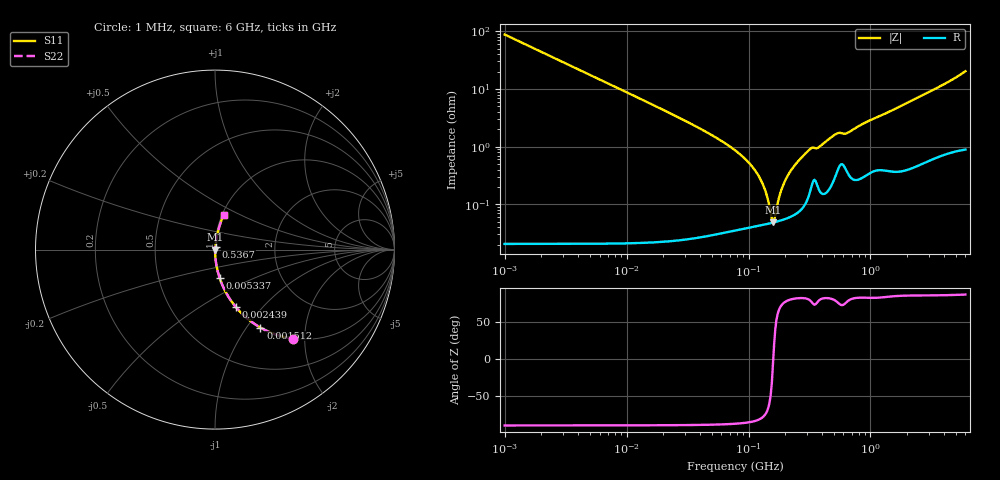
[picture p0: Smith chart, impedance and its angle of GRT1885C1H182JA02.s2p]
!Murata Part Number: GRT1885C1H182JA02
!These Parameters are Measured in Series Mode Connection
!Data Generated on Jun 19, 2026
!  o--ll--o
!Port1  Port2
!  o------o
!Operation Temp=25[degC], DC Bias Voltage=0[V]
!Freq. Start=1000[kHz] Stop=6[GHz] 401[Steps]
# Hz S RI R 50
!Freq.(Hz) S11(Real) S11(Imag) S21(Real) S21(Imag) S12(Real) S12(Imag) S22(Real) S22(Imag)
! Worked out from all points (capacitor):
!   401 points, 1 MHz to 6 GHz, reference 50 ohm
!   read as one part in series: C = 1.81 nF near 1.044 MHz
!   lowest |Z| = 48.4 mohm at 158.8 MHz (marker M1)
!   series resonance near 159.6 MHz, so ESL is about 550 pH
!   S11 on the Smith chart (normalised r, x): 1 MHz: 1.00, -1.76; 1.512 MHz: 1.00, -1.16; 2.439 MHz: 1.00, -0.72; 5.337 MHz: 1.00, -0.33; 536.7 MHz: 1.01, +0.03; 6 GHz: 1.02, +0.41
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1000000  0.4367 -0.4959  0.5633 0.4959  0.5633 0.4959  0.4367 -0.4959
1511688  0.2534 -0.4348  0.7466 0.4348  0.7466 0.4348  0.2534 -0.4348
2439274  0.1154 -0.3192  0.8846 0.3192  0.8846 0.3192  0.1154 -0.3192
4293785  0.0405 -0.1966  0.9595 0.1966  0.9595 0.1966  0.0405 -0.1966
5336962  0.0266 -0.1604  0.9734 0.1604  0.9734 0.1604  0.0266 -0.1604
1.843659e7  0.00243 -0.047  0.9976 0.047  0.9976 0.047  0.00243 -0.047
7.745967e7  0.000423 -0.00863  0.9996 0.00863  0.9996 0.00863  0.000423 -0.00863
1.005588e8  0.000418 -0.00524  0.9996 0.00524  0.9996 0.00524  0.000418 -0.00524
1.223006e8  0.000433 -0.00295  0.9996 0.00295  0.9996 0.00295  0.000433 -0.00295
1.363501e8  0.000449 -0.00173  0.9996 0.00173  0.9996 0.00173  0.000449 -0.00173
1.520136e8  0.00047 -0.000532  0.9995 0.000532  0.9995 0.000532  0.00047 -0.000532
1.587717e8  0.00048 -5.36e-05  0.9995 5.36e-05  0.9995 5.36e-05  0.00048 -5.36e-05
1.658303e8  0.000492 0.000426  0.9995 -0.000426  0.9995 -0.000426  0.000492 0.000426
1.889453e8  0.000536 0.00188  0.9995 -0.00188  0.9995 -0.00188  0.000536 0.00188
2.106508e8  0.000588 0.00313  0.9994 -0.00313  0.9994 -0.00313  0.000588 0.00313
2.561955e8  0.000758 0.00557  0.9992 -0.00557  0.9992 -0.00557  0.000758 0.00557
3.325952e8  0.00233 0.00927  0.9977 -0.00927  0.9977 -0.00927  0.00233 0.00927
3.789555e8  0.00185 0.00965  0.9981 -0.00965  0.9981 -0.00965  0.00185 0.00965
5.366786e8  0.00409 0.0165  0.9959 -0.0165  0.9959 -0.0165  0.00409 0.0165
6.527136e8  0.00369 0.017  0.9963 -0.017  0.9963 -0.017  0.00369 0.017
1.428092e9  0.0053 0.0398  0.9947 -0.0398  0.9947 -0.0398  0.0053 0.0398
6e9  0.0474 0.1918  0.9526 -0.1918  0.9526 -0.1918  0.0474 0.1918
